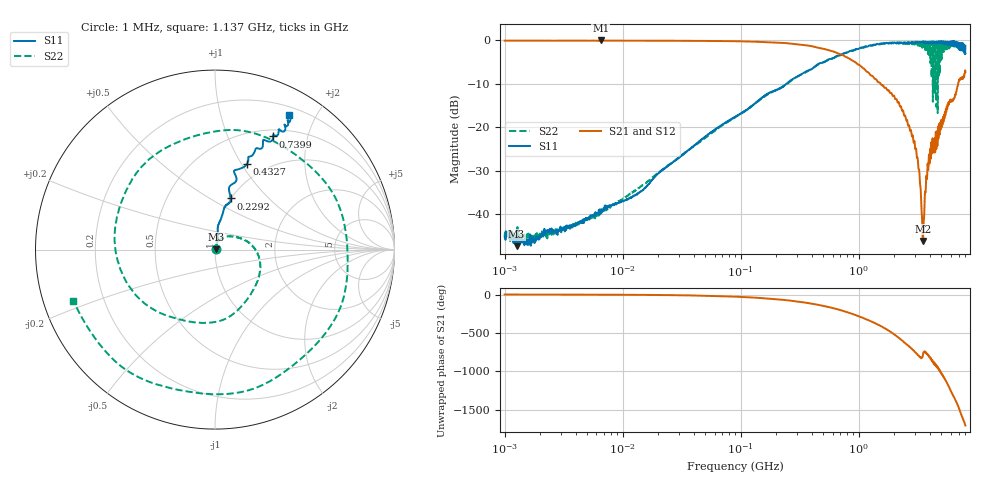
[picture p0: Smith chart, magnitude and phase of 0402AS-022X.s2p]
!s-Parameter Generated by FASTRON Sdn. Bhd.
!FASTRON P/N : 0402AS-022X
!Keysight Technologies: E5071C_MY46733604_B.14.02
!Date: Mon Dec 01 10:32:53 2025
!Version  :Rev00  Mon Dec 01 10:32:53 2025
!Data & Calibration Information:
!Freq  S11:SOLT2(ON)  S21:SOLT2(ON)  S12:SOLT2(ON)  S22:SOLT2(ON)
!PortZ  Port1:50+j0  Port2:50+j0
!When reading reference impedance value at option line is always used.
! Remarks : This data is being provided solely for informational purposes.
# Hz S dB R 50
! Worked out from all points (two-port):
!   1601 points, 1 MHz to 8 GHz, reference 50 ohm
!   highest |S21| = -0.01 dB at 6.532 MHz (marker M1); lowest = -46.1 dB at 3.487 GHz (marker M2)
!   |S21| within 3 dB of the highest: start of sweep to 670 MHz
!   lowest |S11| = -47.3 dB at 1.264 MHz (marker M3), VSWR 1.01, Z = 50.4 + j0.129 ohm
!   |S11| at or under -10 dB: start of sweep to 242.8 MHz
!   |S22| runs from -46.7 to 0.0 dB; largest |S21 - S12| = 0.014
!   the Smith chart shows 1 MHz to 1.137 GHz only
!   S11 on the Smith chart (normalised r, x): 1 MHz: 1.01, +0.00; 229.2 MHz: 1.00, +0.63; 432.7 MHz: 0.82, +1.06; 739.9 MHz: 0.58, +1.48; 1.137 GHz: 0.30, +1.66
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1000000  -45.10 21.4  -0.05 -0.3  -0.04 -0.4  -44.80 21.4
1264032  -47.30 17.3  -0.06 -0.5  -0.04 -0.5  -44.90 5.7
4479405  -41.50 54.3  -0.05 -1.5  -0.05 -1.4  -41.50 53.2
6531720  -39.80 58.9  -0.01 -2.1  -0.05 -2.3  -39.60 62.9
2.00676e7  -30.60 72.1  -0.07 -6.3  -0.07 -6.3  -30.40 70.7
8.994653e7  -17.50 82.8  -0.18 -27.7  -0.18 -27.7  -17.60 32.8
2.292102e8  -10.50 72.8  -0.56 -69.4  -0.56 -69.4  -10.60 -36.9
4.006501e8  -6.56 73.1  -1.33 -120.0  -1.32 -120.0  -6.44 -135.0
4.327027e8  -5.82 69.5  -1.55 -129.0  -1.54 -129.0  -5.87 -150.0
7.399033e8  -2.99 62.8  -3.45 145.0  -3.44 145.0  -3.15 46.9
1.13703e9  -1.35 61.0  -6.81 41.9  -6.81 41.8  -1.52 -160.0
1.349549e9  -0.99 64.0  -8.69 -8.6  -8.71 -8.7  -1.02 95.7
1.542898e9  -0.72 68.6  -10.10 -53.2  -10.10 -53.3  -0.76 1.8
1.7949e9  -0.57 74.2  -11.50 -111.0  -11.50 -112.0  -0.72 -120.0
2.082516e9  -0.54 80.3  -13.50 180.0  -13.50 180.0  -0.72 96.9
2.266813e9  -0.62 82.2  -15.10 136.0  -15.10 136.0  -0.66 7.7
2.457552e9  -0.64 85.8  -17.20 92.4  -17.20 92.3  -0.62 -84.7
2.809687e9  -0.49 95.1  -21.90 12.3  -21.90 12.2  -0.41 101.0
3.183204e9  -0.38 105.0  -28.50 -73.8  -28.50 -74.0  -0.72 -90.2
3.487237e9  -0.35 111.0  -46.10 -71.7  -46.20 -72.4  -0.47 114.0
3.912882e9  -0.66 121.0  -27.10 -72.9  -27.10 -73.6  -0.41 -66.2
8e9  -1.23 -108.0  -7.27 94.5  -7.29 94.1  -2.84 129.0
